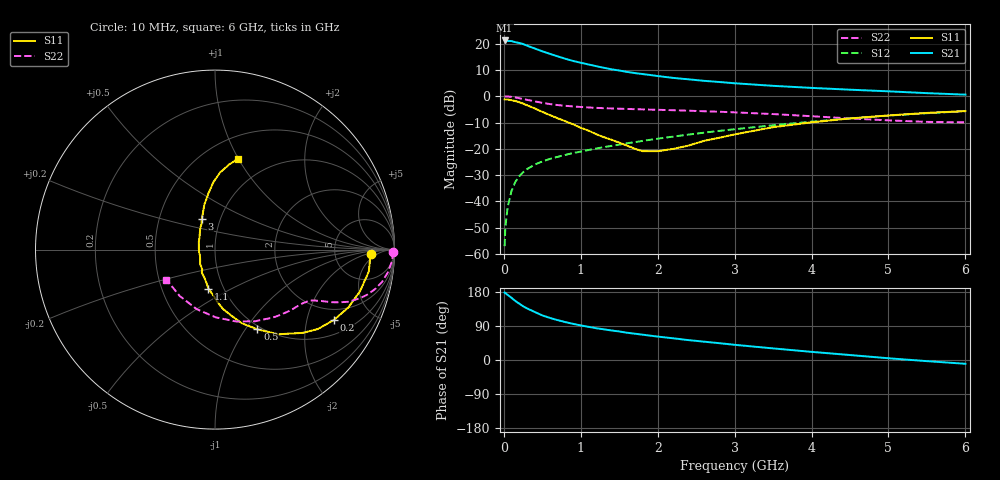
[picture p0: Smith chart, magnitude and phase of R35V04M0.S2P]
! SIEMENS Small Signal Semiconductors
! BFR181
! Si NPN RF Bipolar Junction Transistor in SOT23
! VCE = 5 V  IC = 4 mA
! Common Emitter S-Parameters:  May  1996
# GHz  S  MA  R  50
!  f  S11  S21  S12  S22
! GHz  MAG  ANG  MAG  ANG  MAG  ANG  MAG  ANG
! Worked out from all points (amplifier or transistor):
!   36 points, 10 MHz to 6 GHz, reference 50 ohm
!   highest |S21| = 21.2 dB at 10 MHz (marker M1)
!   |S21| within 3 dB of that: start of sweep to 396.2 MHz
!   unconditionally stable (mu >= 1): 1.257 GHz to 3.11 GHz
!   at 250 MHz: K = 0.36, MSG = 24.4 dB, |S12| = -28.9 dB
!   at 1.4 GHz: K = 1.03, MAG = 13.6 dB, |S12| = -18.9 dB
!   at 6 GHz: K = 0.86, MSG = 3.1 dB, |S12| = -5.7 dB
!   S11 on the Smith chart (normalised r, x): 10 MHz: 14, -3; 200 MHz: 1.52, -2.92; 500 MHz: 0.96, -1.14; 1.1 GHz: 0.85, -0.39; 3 GHz: 0.82, +0.29; 6 GHz: 0.72, +1.00
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0.01  0.8687 -1.8  11.52 178.1  0.0014 91.7  0.9938 -0.7
0.02  0.8659 -3.3  11.33 176.3  0.0033 88.2  0.9917 -1.6
0.05  0.8656 -8.2  11.29 171.8  0.0078 86.4  0.9883 -3.8
0.1  0.8402 -16.1  11.2 164.0  0.0158 82.2  0.9714 -7.5
0.15  0.8102 -23.4  10.68 155.7  0.0235 77.0  0.9479 -11.0
0.2  0.7694 -30.7  10.32 148.8  0.03 73.3  0.9191 -13.8
0.25  0.7238 -37.7  9.849 141.9  0.0357 70.3  0.8862 -16.4
0.3  0.6751 -43.4  9.192 136.3  0.0409 68.8  0.8544 -18.4
0.4  0.5884 -53.3  8.119 126.9  0.0499 65.1  0.8002 -21.3
0.5  0.5031 -62.0  7.161 117.7  0.0573 63.5  0.7485 -23.1
0.6  0.4366 -70.0  6.401 111.0  0.0642 62.0  0.709 -24.4
0.7  0.3806 -75.9  5.739 105.2  0.0703 61.6  0.6791 -25.2
0.8  0.334 -82.3  5.163 100.0  0.0765 61.0  0.6571 -25.8
0.9  0.2916 -87.4  4.694 95.4  0.0829 60.9  0.6395 -26.5
1.1  0.2218 -99.4  4.025 87.6  0.0946 61.8  0.6112 -27.6
1.6  0.115 -136.4  2.905 72.0  0.1272 62.2  0.5729 -31.5
2.2  0.0992 155.5  2.233 57.3  0.1704 61.3  0.542 -38.3
3  0.1877 112.8  1.766 40.1  0.2355 57.5  0.4934 -50.4
3.5  0.2576 103.3  1.577 30.6  0.2802 53.8  0.4574 -60.8
4.5  0.3776 91.2  1.332 13.1  0.3779 44.1  0.3777 -89.3
5.5  0.4813 80.5  1.145 -3.0  0.4749 31.7  0.3248 -127.3
6  0.5215 75.8  1.072 -10.0  0.5196 24.7  0.3182 -148.4
